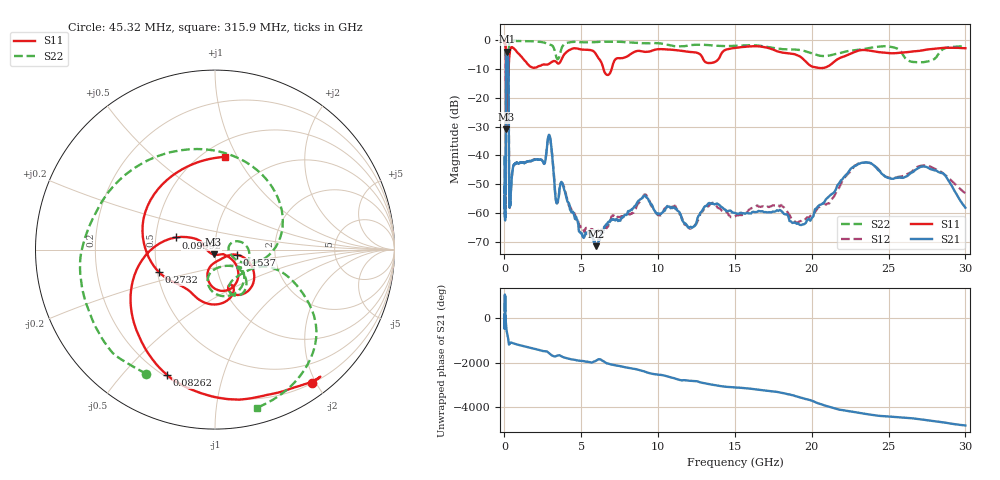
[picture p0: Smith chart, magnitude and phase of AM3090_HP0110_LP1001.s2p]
! Date/Time: Thu, Feb 28, 2019 2:00 PM
! Network Analyzer: Agilent Technologies E8364B Rev: A.07.50.67
! Sweep from 0.010 to 30.000 GHz, 1601 Points, Sweep Type: LOG
! Power Supply: 5.023 V, 0.002 A
# Hz S DB R 50
!freq MagS11 AngS11 MagS21 AngS21 MagS12 AngS12 MagS22 AngS22
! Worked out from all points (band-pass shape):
!   1601 points, 10 MHz to 30 GHz, reference 50 ohm
!   highest |S21| = -4.06 dB at 159.1 MHz (marker M1); lowest = -71.5 dB at 5.959 GHz (marker M2)
!   |S21| within 3 dB of the highest: 111.1 MHz to 250 MHz (138.9 MHz wide, 76.9 % of centre)
!   lowest |S11| = -31.0 dB at 107.7 MHz (marker M3), VSWR 1.06, Z = 49.1 - j2.66 ohm
!   |S11| at or under -10 dB: 98.36 MHz to 270 MHz (171.6 MHz wide, 93.2 % of centre); 6.447 GHz to 6.978 GHz (530.6 MHz wide, 7.9 % of centre)
!   |S22| runs from -22.4 to -0.1 dB; largest |S21 - S12| = 0.018
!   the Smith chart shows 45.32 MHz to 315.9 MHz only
!   S11 on the Smith chart (normalised r, x): 45.32 MHz: 0.20, -1.95; 82.62 MHz: 0.21, -0.67; 99.92 MHz: 0.64, +0.09; 153.7 MHz: 1.28, -0.08; 273.2 MHz: 0.51, -0.14; 315.9 MHz: 0.63, +0.89
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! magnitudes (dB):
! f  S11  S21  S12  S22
! 10 MHz  -0.3  -40.5  -40.4  -0.7
! 38.04 MHz  -0.5  -59.6  -57.1  -1.5
! 45.32 MHz  -0.7  -52.7  -53.7  -2.0
! 82.62 MHz  -2.5  -50.3  -52.8  -4.8
! 99.92 MHz  -12.8  -16.2  -16.1  -11.6
! 107.7 MHz  -31.0  -8.3  -8.3  -22.0
! 123.3 MHz  -12.6  -5.4  -5.3  -15.1
! 144.7 MHz  -24.1  -4.3  -4.2  -15.9
! 153.7 MHz  -17.9  -4.1  -4.0  -15.3
! 159.1 MHz  -14.1  -4.1  -4.0  -14.1
! 244.7 MHz  -10.9  -6.5  -6.5  -11.8
! 273.2 MHz  -9.5  -16.4  -16.3  -7.9
! 315.9 MHz  -5.7  -57.2  -56.3  -0.8
! 550.5 MHz  -2.7  -44.4  -44.5  -0.2
! 2.084 GHz  -9.5  -41.4  -41.3  -0.5
! 2.928 GHz  -8.2  -33.0  -32.9  -1.6
! 3.402 GHz  -7.7  -56.6  -56.6  -6.3
! 5.959 GHz  -4.9  -71.5  -66.7  -0.7
! 7.926 GHz  -5.8  -60.7  -60.8  -0.7
! 19.31 GHz  -6.0  -64.2  -62.8  -3.5
! 23.36 GHz  -3.4  -42.6  -42.6  -3.1
! 30 GHz  -2.8  -58.2  -53.1  -2.2
